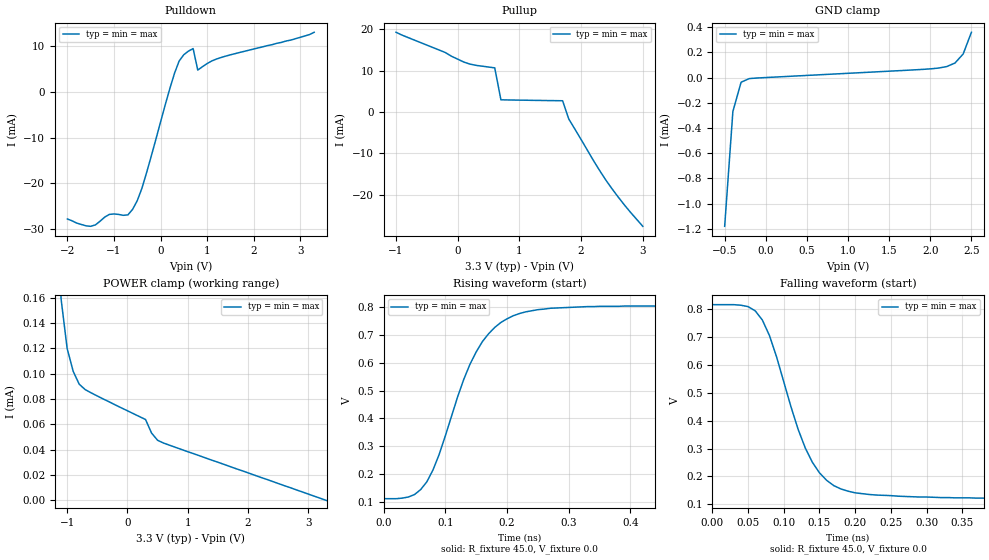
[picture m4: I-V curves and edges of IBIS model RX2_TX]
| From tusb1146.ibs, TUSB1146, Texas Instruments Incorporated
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[Model] RX2_TX
Model_type Output
| typ min max
C_comp 0.268p 0.268p 0.268p
[Algorithmic Model]
Executable Windows_cl19.00.24215.1_64  RX2_TX_x64.dll RX2_TX.ami
Executable Linux_gcc5.4.0_64 RX2_TX_x64.so RX2_TX.ami
[End Algorithmic Model]
[Temperature_Range] 27 27 27
[Voltage Range] 3.3 3.3 3.3
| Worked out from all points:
|   slope of the pulldown table from 0 to 0.495 V, typ, clamps not added: 33.8 ohm
|   slope of the pullup table from 0 to 0.495 V, typ, clamps not added: 262 ohm
|   GND clamp passes 1 mA (typ) near -0.48 V on its own axis
|   POWER clamp passes 1 mA (typ) near -1.34 V on its own axis
|   rising waveform, R_fixture 45.0, V_fixture 0.0: 20-80 % time 71.8ps typ, 71.8ps min, 71.8ps max; typ from 0.111 V to 0.81 V
|   falling waveform, R_fixture 45.0, V_fixture 0.0: 20-80 % time 54.7ps typ, 54.7ps min, 54.7ps max; typ from 0.817 V to 0.12 V
[GND_clamp]
|   Voltage   I(typ)   I(min)   I(max)
-500mV    -1.18mA    -1.18mA    -1.18mA
-400mV    -269uA     -269uA     -269uA
-300mV    -36.9uA    -36.9uA    -36.9uA
-200mV    -8.18uA    -8.18uA    -8.18uA
1.9V      64.4uA     64.4uA     64.4uA
2.2V      87.1uA     87.1uA     87.1uA
2.3V      115uA      115uA      115uA
2.4V      187uA      187uA      187uA
2.5V      359uA      359uA      359uA
[Power_clamp]
| Note that the[POWER_clamp]voltage table is referenced to Vcc
| and is calculated using Vtable=Vcc - Vmeasured.
|   Voltage   I(typ)   I(min)   I(max)
-1.7V     31.1mA     31.1mA     31.1mA
-1.1V     159uA      159uA      159uA
-1V       120uA      120uA      120uA
-900mV    102uA      102uA      102uA
-800mV    91.8uA     91.8uA     91.8uA
-700mV    87.5uA     87.5uA     87.5uA
-600mV    84.9uA     84.9uA     84.9uA
300mV     63.9uA     63.9uA     63.9uA
400mV     53.2uA     53.2uA     53.2uA
500mV     47.5uA     47.5uA     47.5uA
1V        38.5uA     38.5uA     38.5uA
3.3V      -18.2pA    -18.2pA    -18.2pA
[Pulldown]
|   Voltage   I(typ)   I(min)   I(max)
-2V       -27.8mA    -27.8mA    -27.8mA
-1.5V     -29.4mA    -29.4mA    -29.4mA
-1.1V     -26.8mA    -26.8mA    -26.8mA
-600mV    -25.7mA    -25.7mA    -25.7mA
-400mV    -21.1mA    -21.1mA    -21.1mA
300mV     4.04mA     4.04mA     4.04mA
400mV     6.72mA     6.72mA     6.72mA
600mV     8.88mA     8.88mA     8.88mA
700mV     9.44mA     9.44mA     9.44mA
800mV     4.74mA     4.74mA     4.74mA
1.3V      7.49mA     7.49mA     7.49mA
3.3V      13mA       13mA       13mA
[Pullup]
|   Voltage   I(typ)   I(min)   I(max)
| Note that the[Pullup]voltage table is referenced to Vcc
| and is calculated using Vtable=Vcc - Vmeasured.
-1V       19.3mA     19.3mA     19.3mA
-200mV    14.4mA     14.4mA     14.4mA
100mV     12.1mA     12.1mA     12.1mA
300mV     11.3mA     11.3mA     11.3mA
600mV     10.7mA     10.7mA     10.7mA
700mV     2.98mA     2.98mA     2.98mA
1.7V      2.75mA     2.75mA     2.75mA
1.8V      -1.66mA    -1.66mA    -1.66mA
2.3V      -14.1mA    -14.1mA    -14.1mA
2.4V      -16.4mA    -16.4mA    -16.4mA
2.6V      -20.5mA    -20.5mA    -20.5mA
3V        -27.6mA    -27.6mA    -27.6mA
[Ramp]
|   typ   min   max
dV/dt_r   0.42/71p 0.42/71p 0.42/71p
dV/dt_f   0.42/52p 0.42/52p 0.42/52p
R_load = 45ohm | Note: Measurement is single ended with 25ohm to ground
[Rising Waveform]
R_fixture = 45.0
V_fixture = 0.0
V_fixture_min = 0.0
V_fixture_max = 0.0
C_fixture = 0p
L_fixture = 0n
|   V(typ)   V(min)   V(max)
0s        111mV      111mV      111mV
40ps      117mV      117mV      117mV
70ps      172mV      172mV      172mV
90ps      271mV      271mV      271mV
140ps     596mV      596mV      596mV
160ps     677mV      677mV      677mV
180ps     728mV      728mV      728mV
230ps     784mV      784mV      784mV
330ps     803mV      803mV      803mV
9.9ns     810mV      810mV      810mV
[Falling Waveform]
R_fixture = 45.0
V_fixture = 0.0
V_fixture_min = 0.0
V_fixture_max = 0.0
C_fixture = 0p
L_fixture = 0n
|   V(typ)   V(min)   V(max)
0s        817mV      817mV      817mV
50ps      810mV      810mV      810mV
70ps      762mV      762mV      762mV
80ps      706mV      706mV      706mV
120ps     370mV      370mV      370mV
130ps     303mV      303mV      303mV
160ps     186mV      186mV      186mV
200ps     141mV      141mV      141mV
290ps     126mV      126mV      126mV
9.9ns     120mV      120mV      120mV
